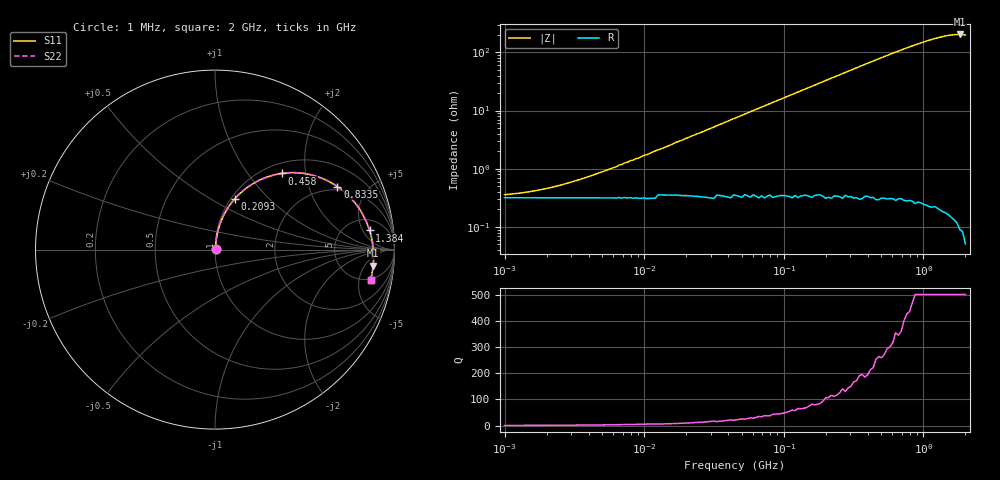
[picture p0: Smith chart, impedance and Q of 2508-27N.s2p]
# MHz S MA R 50
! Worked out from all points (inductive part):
!   166 points, 1 MHz to 2 GHz, reference 50 ohm
!   read as one part in series: L = 26.3 nH near 5.758 MHz
!   highest |Z| = 203 ohm at 1.824 GHz (marker M1)
!   S11 on the Smith chart (normalised r, x): 1 MHz: 1.01, +0.00; 209.3 MHz: 1.04, +0.65; 458 MHz: 1.19, +1.49; 833.5 MHz: 1.84, +3.13; 1.384 GHz: 8, +7; 2 GHz: 4.76, -7.30
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1  0.003664 24.5  0.997 -0.1  0.997 -0.1  0.003665 24.5
1.906  0.004421 40.9  0.997 -0.2  0.997 -0.2  0.004423 40.9
3.632  0.006464 58.6  0.997 -0.4  0.997 -0.4  0.006469 58.6
6.313  0.01 70.3  0.997 -0.6  0.997 -0.6  0.01 70.3
7.249  0.012 72.5  0.997 -0.7  0.997 -0.7  0.012 72.5
9.126  0.014 75.6  0.997 -0.9  0.997 -0.9  0.014 75.6
10.007  0.016 76.7  0.997 -1.0  0.997 -1.0  0.016 76.7
10.479  0.016 77.2  0.997 -1.1  0.997 -1.1  0.016 77.2
12.599  0.019 78.9  0.996 -1.3  0.996 -1.3  0.02 78.9
13.193  0.02 79.3  0.996 -1.3  0.996 -1.3  0.02 79.3
45.763  0.07 82.6  0.994 -4.6  0.994 -4.6  0.07 82.6
91.33  0.138 79.4  0.987 -9.2  0.987 -9.2  0.138 79.4
166.224  0.245 72.7  0.966 -16.6  0.966 -16.6  0.245 72.7
209.278  0.303 68.8  0.95 -20.7  0.95 -20.7  0.303 68.8
316.796  0.432 59.4  0.899 -30.2  0.899 -30.2  0.433 59.4
457.963  0.566 48.6  0.822 -41.1  0.822 -41.1  0.567 48.6
576.582  0.65 40.8  0.757 -49.0  0.757 -49.0  0.651 40.8
833.511  0.767 27.2  0.639 -62.7  0.639 -62.7  0.768 27.2
1049.404  0.823 18.3  0.566 -71.6  0.566 -71.6  0.824 18.3
1383.503  0.868 7.0  0.495 -82.9  0.495 -82.9  0.869 7.0
1823.969  0.885 -5.9  0.462 -95.8  0.462 -95.8  0.886 -5.9
2000  0.883 -11.0  0.467 -101.0  0.467 -101.0  0.884 -11.0
